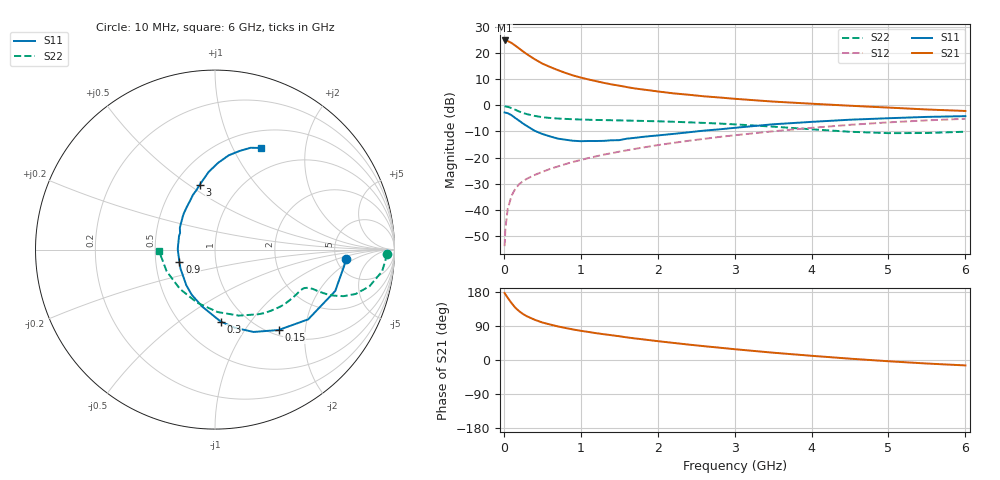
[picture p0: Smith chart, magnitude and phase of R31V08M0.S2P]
! SIEMENS Small Signal Semiconductors
! BFR181
! Si NPN RF Bipolar Junction Transistor in SOT23
! VCE = 1 V  IC = 8 mA
! Common Emitter S-Parameters:  May  1996
# GHz  S  MA  R  50
!  f  S11  S21  S12  S22
! GHz  MAG  ANG  MAG  ANG  MAG  ANG  MAG  ANG
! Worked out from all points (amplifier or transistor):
!   36 points, 10 MHz to 6 GHz, reference 50 ohm
!   highest |S21| = 24.9 dB at 10 MHz (marker M1)
!   |S21| within 3 dB of that: start of sweep to 195.6 MHz
!   unconditionally stable (mu >= 1): 555.9 MHz to 3.341 GHz
!   at 250 MHz: K = 0.65, MSG = 24.9 dB, |S12| = -29.0 dB
!   at 1.4 GHz: K = 1.18, MAG = 10.6 dB, |S12| = -18.3 dB
!   at 6 GHz: K = 0.95, MSG = 1.5 dB, |S12| = -5.1 dB
!   S11 on the Smith chart (normalised r, x): 10 MHz: 6.13, -1.38; 150 MHz: 1.09, -1.45; 300 MHz: 0.76, -0.73; 900 MHz: 0.66, -0.10; 3 GHz: 0.66, +0.55; 6 GHz: 0.70, +1.30
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0.01  0.7314 -4.1  17.55 176.8  0.002 86.3  0.9601 -1.4
0.02  0.7248 -7.4  17.34 173.5  0.0043 87.3  0.9536 -3.0
0.05  0.7084 -19.0  17.12 164.3  0.0103 79.7  0.939 -7.4
0.1  0.6486 -36.8  15.72 150.2  0.0185 72.8  0.8843 -13.4
0.15  0.571 -51.7  13.94 137.8  0.0254 67.6  0.8219 -17.5
0.2  0.5063 -65.0  12.29 128.7  0.0309 65.0  0.762 -19.9
0.25  0.4483 -75.9  10.8 121.2  0.0353 62.7  0.7131 -21.1
0.3  0.402 -85.5  9.568 115.4  0.0392 62.1  0.6792 -21.7
0.4  0.3259 -102.5  7.681 106.3  0.0463 62.0  0.6278 -22.0
0.5  0.283 -117.3  6.331 99.0  0.0531 63.0  0.5937 -21.9
0.6  0.2545 -129.0  5.451 93.7  0.0604 63.7  0.5741 -22.0
0.7  0.2309 -140.3  4.752 88.8  0.0673 64.6  0.5594 -22.4
0.9  0.2098 -160.9  3.744 80.6  0.0825 65.8  0.542 -23.3
1.1  0.2075 179.6  3.138 74.0  0.0978 66.7  0.5301 -25.1
1.3  0.2087 166.4  2.698 68.0  0.1138 67.0  0.5221 -27.1
1.6  0.2301 148.3  2.24 59.7  0.1378 66.2  0.5116 -31.0
2.2  0.2834 124.0  1.703 45.2  0.1906 63.5  0.4854 -40.4
3  0.3711 103.3  1.337 28.5  0.2672 57.2  0.4327 -56.4
3.5  0.4339 94.7  1.182 19.3  0.3186 52.3  0.3909 -70.2
4.5  0.5311 81.7  0.984 3.5  0.4236 39.9  0.3118 -108.7
5.5  0.6012 70.7  0.834 -9.3  0.5157 25.8  0.2953 -155.9
6  0.6216 65.6  0.781 -14.3  0.5538 18.2  0.3127 -178.9
